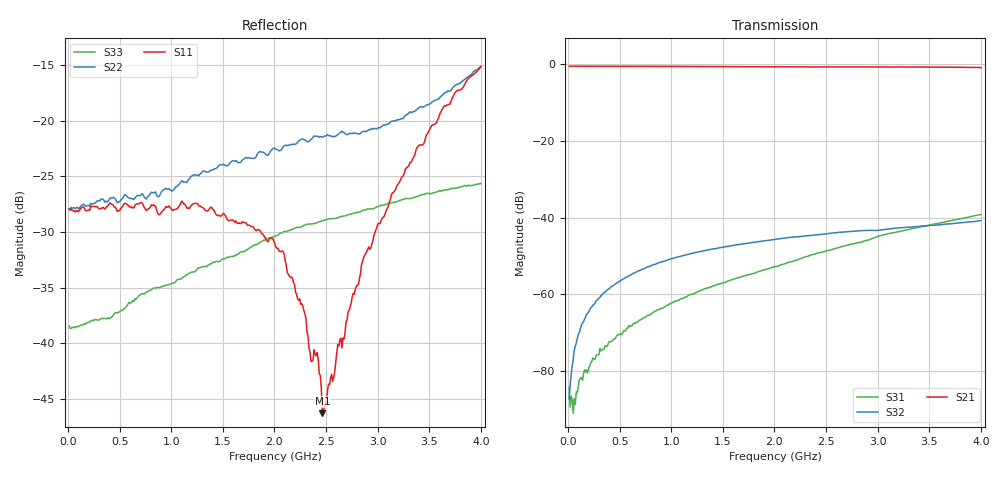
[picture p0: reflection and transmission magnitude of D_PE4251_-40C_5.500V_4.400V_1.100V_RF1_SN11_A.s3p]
! Device ID: PE4251_SoldCshunt_081809
! Dir: c:\Test Bench Repositories\Bench_Software_CVI_Version_8\trunk\PSC 4Port_VNA Bench\datalog\4250\TEST\PE4251_SoldCshunt_081809\-40C\5p500000\RF1
! Serial: 11
! Insertion: A
! Temp: -40C
! VDD: 5.500
! Control_Hi: 80.000
! Control_Lo: 20.000
! Logic State: RF1
! Port 1: RFC
! Port 2: RF1
! Port 3: RF2
! V1 = 1.10
! V2 = 4.40
! V3 = 1.10
! IDD: 6.318720e-05
! FILE NAME
! DATE 08/18/09  20:10
! CORRECTED  DATA
#  Hz  S  RI  R  50.00
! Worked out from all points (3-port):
!   401 points, 10 MHz to 4 GHz, reference 50 ohm
!   strongest paths, dB at 10 MHz, 1.008 GHz, 2.005 GHz, 3.002 GHz, 4 GHz:
!     S21: -0.5, -0.5, -0.6, -0.7, -0.9
!     S32: -87.2, -50.6, -45.6, -43.3, -40.7
!     S31: -84.3, -62.2, -52.8, -44.8, -39.2
!   lowest |S11| = -46.3 dB at 2.464 GHz (marker M1), VSWR 1.01, Z = 50.2 - j0.462 ohm
!   |S11| at or under -10 dB: start of sweep to end of sweep
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1e7  0.0402 0.000136  0.9448 -0.0026  3.67e-05 2.83e-05
     0.9452 -0.00445  0.0402 4.94e-05  0.000109 3.34e-05
     -6.68e-06 -6.08e-05  2.41e-05 -3.62e-05  0.012 -0.000352
1.0975e8  0.0395 0.000425  0.9451 -0.0379  4.79e-06 -7.47e-05
          0.9451 -0.0381  0.0405 0.000219  3.47e-05 0.000326
          -5.67e-06 -7.9e-05  1.73e-05 0.000319  0.012 0.000837
1.8955e8  0.0395 0.0005  0.943 -0.0645  -1.37e-06 -0.000113
          0.9425 -0.0647  0.0416 1.67e-05  4.81e-05 0.000569
          -8.41e-06 -9.42e-05  4.03e-05 0.000567  0.0123 0.00164
4.888e8  0.0394 -0.00283  0.929 -0.1631  -0.000156 -0.000259
         0.9286 -0.1624  0.0432 -0.00291  0.000137 0.00144
         -0.00016 -0.000255  0.000137 0.00145  0.0132 0.00391
1.0474e9  0.0378 -0.0132  0.878 -0.3377  -0.000709 -0.000419
          0.8784 -0.3371  0.049 -0.0124  0.000534 0.003
          -0.000703 -0.000423  0.000531 0.00299  0.0161 0.0102
2.005e9  0.026 -0.0102  0.7216 -0.5846  -0.00226 -0.000455
         0.7217 -0.5847  0.0662 -0.0356  0.00122 0.00508
         -0.00226 -0.000459  0.00122 0.00508  0.0185 0.0238
2.2843e9  0.0108 -0.009  0.6658 -0.6446  -0.00299 -0.000547
          0.6643 -0.6453  0.0644 -0.0511  0.00138 0.00558
          -0.003 -0.000552  0.00138 0.00559  0.0172 0.0292
2.46385e9  0.00152 -0.0046  0.629 -0.6798  -0.00351 -0.000475
           0.628 -0.6799  0.0613 -0.058  0.00138 0.00592
           -0.00352 -0.000501  0.00139 0.00594  0.0156 0.032
3.14215e9  -0.0366 -0.0301  0.4626 -0.8016  -0.00633 -1.56e-05
           0.4648 -0.7993  0.022 -0.0971  0.00119 0.00713
           -0.00634 -3.41e-05  0.00121 0.00713  0.00725 0.0421
4e9  -0.1567 -0.0772  0.1819 -0.8907  -0.0108 0.00217
     0.1819 -0.8877  -0.1203 -0.1284  7.18e-05 0.00918
     -0.0108 0.00213  5.33e-05 0.00919  -0.0133 0.0504
